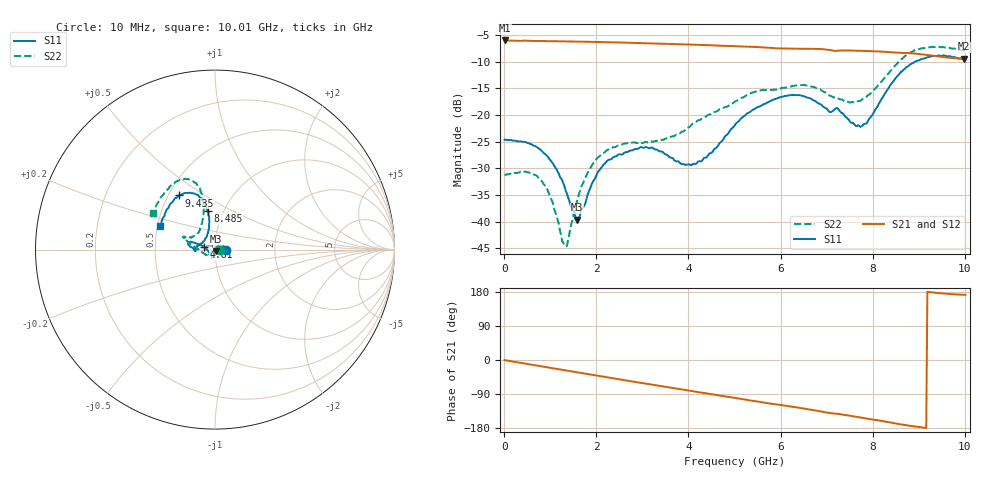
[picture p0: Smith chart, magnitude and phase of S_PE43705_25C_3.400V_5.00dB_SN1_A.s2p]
! Device ID: PE43705
! Serial: 1
! Insertion: A
! Impedance: 50 ohm
! Temp: 25C
! VDD: 3.400V
! Attenuation Step: 5.00dB
#  Hz  S  RI  R  50
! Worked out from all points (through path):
!   401 points, 10 MHz to 10.01 GHz, reference 50 ohm
!   highest |S21| = -6.02 dB at 10 MHz (marker M1); lowest = -9.4 dB at 9.985 GHz (marker M2)
!   group delay of S21, straight-line fit = 53.6 ps
!   lowest |S11| = -39.7 dB at 1.585 GHz (marker M3), VSWR 1.02, Z = 50.8 - j0.716 ohm
!   |S11| at or under -10 dB: start of sweep to 8.917 GHz
!   |S22| runs from -44.6 to -7.2 dB; largest |S21 - S12| = 0.0044
!   S11 on the Smith chart (normalised r, x): 10 MHz: 1.12, -0.00; 4.81 GHz: 0.88, +0.03; 8.485 GHz: 0.84, +0.38; 9.435 GHz: 0.57, +0.39; 10.01 GHz: 0.52, +0.15
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1e7  0.0587 -8.65e-05  0.5003 -0.00241  0.5008 -0.00219  0.0276 3.45e-05
7.85e8  0.0436 0.0186  0.4746 -0.1385  0.4746 -0.1383  0.0168 0.018
1.01e9  0.0343 0.0151  0.4602 -0.1761  0.4601 -0.1758  0.00931 0.014
1.31e9  0.0206 0.00533  0.4373 -0.2221  0.4374 -0.2219  -0.00325 0.00489
1.385e9  0.017 0.00184  0.4306 -0.2335  0.4308 -0.2334  -0.00627 0.00186
1.585e9  0.00761 -0.00705  0.4113 -0.2624  0.4115 -0.2623  -0.0141 -0.00688
1.685e9  0.00389 -0.0126  0.4014 -0.2762  0.4014 -0.2761  -0.0186 -0.0114
1.96e9  -0.00556 -0.0241  0.3709 -0.3122  0.3709 -0.3117  -0.0288 -0.0221
2.235e9  -0.0114 -0.0353  0.337 -0.3444  0.3372 -0.3442  -0.0358 -0.0305
3.36e9  -0.0159 -0.0431  0.1753 -0.4329  0.1757 -0.4325  -0.049 -0.0293
4.11e9  -0.0303 -0.0167  0.058 -0.4535  0.0588 -0.4531  -0.0829 -0.00853
4.81e9  -0.062 0.016  -0.0493 -0.4419  -0.0485 -0.442  -0.1177 0.0179
5.01e9  -0.0769 0.025  -0.0784 -0.4344  -0.0777 -0.4349  -0.1308 0.0272
5.96e9  -0.1386 0.0437  -0.1987 -0.373  -0.1974 -0.373  -0.1643 0.0618
6.685e9  -0.1382 0.0168  -0.2777 -0.3112  -0.2778 -0.3113  -0.1688 0.0724
7.735e9  -0.0596 0.0494  -0.3528 -0.1895  -0.3514 -0.1904  -0.0852 0.1062
8.36e9  -0.0331 0.1817  -0.375 -0.1046  -0.3736 -0.1064  -0.0641 0.2445
8.485e9  -0.0403 0.2153  -0.3762 -0.0858  -0.3749 -0.0881  -0.0686 0.2832
8.91e9  -0.0919 0.3013  -0.3758 -0.0309  -0.3735 -0.0316  -0.1262 0.3846
9.435e9  -0.1995 0.3019  -0.3525 0.0215  -0.3517 0.0218  -0.2248 0.3728
9.985e9  -0.2997 0.1387  -0.3347 0.0466  -0.3355 0.0457  -0.3372 0.2129
1.001e10  -0.307 0.1293  -0.3356 0.0475  -0.3369 0.0464  -0.3451 0.2014
